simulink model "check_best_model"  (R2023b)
settings: Solver=VariableStepAuto  StartTime=0.0  StopTime=10.0  RelTol=1e-3
libraries: slident x1

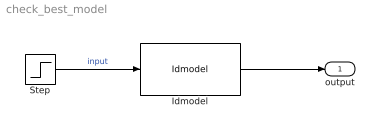
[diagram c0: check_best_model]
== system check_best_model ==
  Idmodel : slident/Models/Idmodel  sys=best_model  IC=0  noi=off  seed=[]
  Step : Step  After=5  SampleTime=0
  output : Outport
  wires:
  Step/1 -> Idmodel/1  "input"
  Idmodel/1 -> output/1
